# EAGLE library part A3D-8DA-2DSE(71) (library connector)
HIROSE(HRS) - A3D-8DA-2DSE(71) - CONNECTOR, RCPT, 8POS, 2ROW, 2MM Source: Datasheet
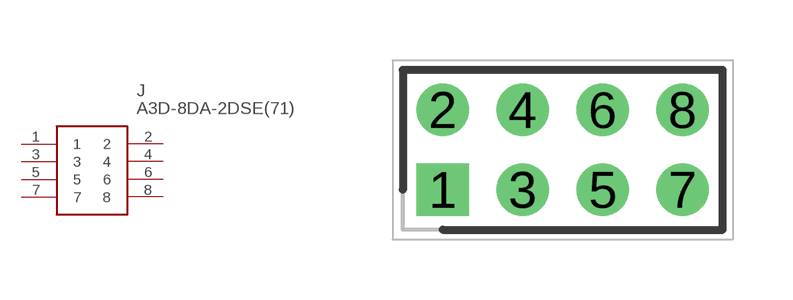
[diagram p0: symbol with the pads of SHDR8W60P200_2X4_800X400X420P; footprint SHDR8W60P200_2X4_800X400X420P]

Designator prefix J

## A3D-8DA-2DSE(71) (DESCRIPTION: HIROSE(HRS) - A3D-8DA-2DSE(71) - CONNECTOR, RCPT, 8POS, 2ROW, 2MM; HEIGHT: 4.2mm; MANUFACTURER_NAME: Hirose; MANUFACTURER_PART_NUMBER: A3D-8DA-2DSE(71); MOUSER_PART_NUMBER: 798-A3D-8DA-2DSE71; MOUSER_PRICE-STOCK: https://www.mouser.com/Search/Refine.aspx?Keyword=798-A3D-8DA-2DSE71)  [SHDR8W60P200_2X4_800X400X420P]
1  1
2  2
3  3
4  4
5  5
6  6
7  7
8  8

## Footprint SHDR8W60P200_2X4_800X400X420P (pad centres in mm)
A3D-8DA-2DSE(71)
drill 0.8 pad 1.2 square: 1 0,0
drill 0.8 pad 1.2: 2 0,2; 3 2,0; 4 2,2; 5 4,0; 6 4,2; 7 6,0; 8 6,2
